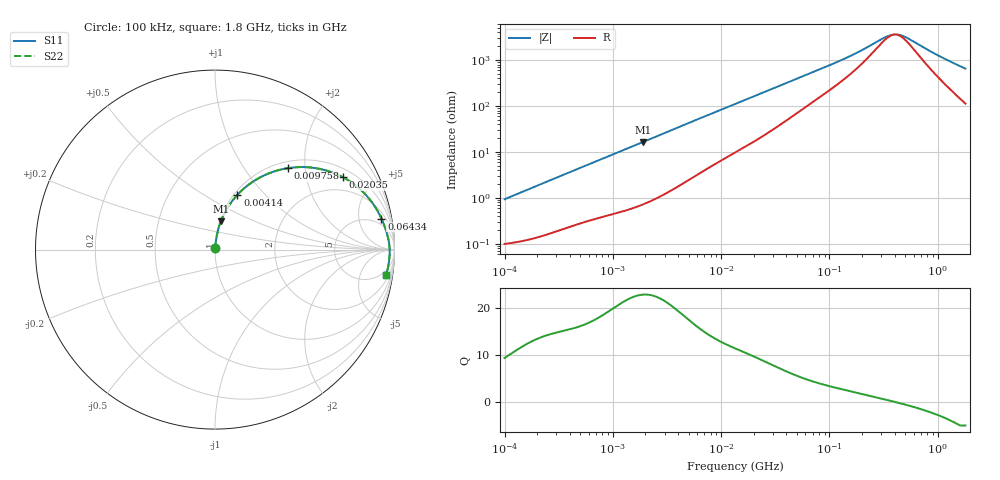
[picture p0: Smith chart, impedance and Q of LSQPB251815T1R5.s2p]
! LSQPB251815T1R5  S-PARAMETER MODEL  ( General Type )
! Model Generated by TAIYO YUDEN Corporation (http://www.ty-top.com)
! Version 2.0
! TAIYO YUDEN Control No. 110926NG22SB-FKC
! Copyright(c) 2010 TAIYO YUDEN CO.,LTD. All Rights Reserved.
! Product Description (link to TY-COMPAS)
! https://ds.yuden.co.jp/TYCOMPAS/or/detail?pn=LSQPB251815T1R5M&u=M
! Products Name : Inductors
! Characteristics :
!  Inductance : 1.5 uH , SRF(min) : 350 MHz , DC Resistance(max) : 0.1105 Ohm
!  Rated Current : Saturation :1700 mA , Temp Rise : 1100 mA (40 degC)
!  Case Size : 2.5 x 1.8 / 0.098 x 0.071 [mm/inch] , Thickness : 1.5 / 0.06 [mm/inch]
!  (Conditions: Temperature = 25 degC , DC Bias Current/Voltage = 0A / 0V)
! External Node Assignments :
!  1  o---GGG---o  2
! GND o---------o GND
! Frequency Range : 0.1MHz  -  1800MHz  [ 402 STEP ]
# MHz S RI R 50
! Freq[MHz].  S11 Real  S11 Imag  S21 Real  S21 Imag  S12 Real  S12 Imag  S22 Real  S22 Imag
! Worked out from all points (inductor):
!   401 points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, 100 kHz to 1.8 GHz, reference 50 ohm
!   read as one part in series: L = 1.48 uH near 105 kHz
!   highest Q = 22.8 at 1.891 MHz (marker M1), where L = 1.38 uH
!   self-resonance near 402.1 MHz
!   S11 on the Smith chart (normalised r, x): 100 kHz: 1.00, +0.02; 4.14 MHz: 1.04, +0.71; 9.758 MHz: 1.13, +1.63; 20.35 MHz: 1.34, +3.29; 64.34 MHz: 3, +10; 1.8 GHz: 3, -13
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0.1  0.00108 0.00931  0.9989 -0.00931  0.9989 -0.00931  0.00108 0.00931
0.516129  0.00498 0.046  0.995 -0.046  0.995 -0.046  0.00498 0.046
1.050184  0.0129 0.0907  0.9871 -0.0907  0.9871 -0.0907  0.0129 0.0907
1.890522  0.0329 0.1578  0.9671 -0.1578  0.9671 -0.1578  0.0329 0.1578
2.66389  0.0593 0.2146  0.9407 -0.2146  0.9407 -0.2146  0.0593 0.2146
4.140031  0.1249 0.3053  0.8751 -0.3053  0.8751 -0.3053  0.1249 0.3053
6.278453  0.2357 0.3937  0.7643 -0.3937  0.7643 -0.3937  0.2357 0.3937
9.75753  0.4068 0.4539  0.5932 -0.4539  0.5932 -0.4539  0.4068 0.4539
13.41641  0.5468 0.4558  0.4532 -0.4558  0.4532 -0.4558  0.5468 0.4558
20.3463  0.7127 0.4033  0.2873 -0.4033  0.2873 -0.4033  0.7127 0.4033
25.99364  0.7883 0.3537  0.2117 -0.3537  0.2117 -0.3537  0.7883 0.3537
34.03197  0.8499 0.2945  0.1501 -0.2945  0.1501 -0.2945  0.8499 0.2945
64.33982  0.9274 0.1731  0.0726 -0.1731  0.0726 -0.1731  0.9274 0.1731
69.24595  0.9324 0.1619  0.0676 -0.1619  0.0676 -0.1619  0.9324 0.1619
155.4012  0.9634 0.0695  0.0366 -0.0695  0.0366 -0.0695  0.9634 0.0695
208.5031  0.9683 0.0456  0.0317 -0.0456  0.0317 -0.0456  0.9683 0.0456
308.5485  0.972 0.0177  0.028 -0.0177  0.028 -0.0177  0.972 0.0177
357.3983  0.9728 0.00782  0.0272 -0.00782  0.0272 -0.00782  0.9728 0.00782
413.9822  0.9732 -0.00193  0.0268 0.00193  0.0268 0.00193  0.9732 -0.00193
491.4156  0.9733 -0.0135  0.0267 0.0135  0.0267 0.0135  0.9733 -0.0135
1024.694  0.9688 -0.0719  0.0312 0.0719  0.0312 0.0719  0.9688 -0.0719
1800  0.9538 -0.1397  0.0462 0.1397  0.0462 0.1397  0.9538 -0.1397
